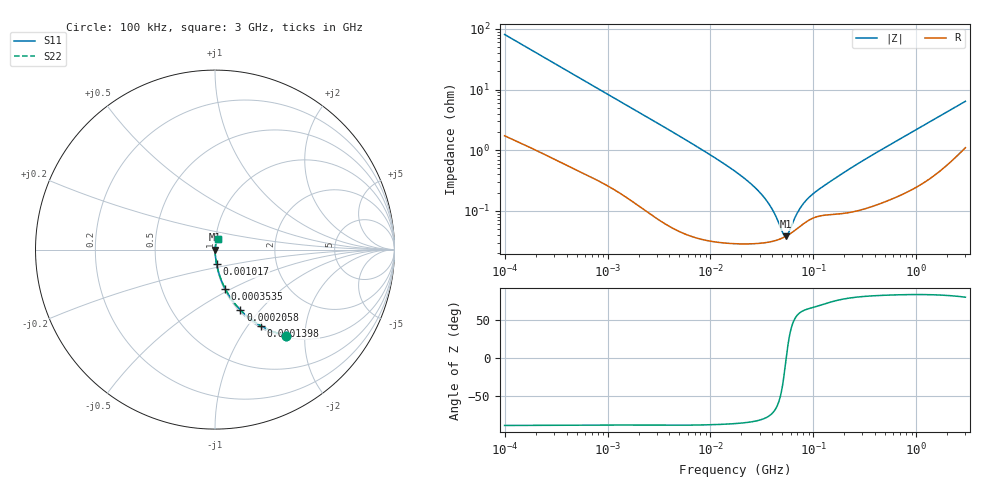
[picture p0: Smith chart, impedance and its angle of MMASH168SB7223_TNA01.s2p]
! MMASH168SB7223_TNA01  S-PARAMETER MODEL  ( Standard Model )
! Model Generated by TAIYO YUDEN Corporation (http://www.ty-top.com)
! Version 1.0
! TAIYO YUDEN Control No. 220601
! Copyright(c) 2013 TAIYO YUDEN CO.,LTD. All Rights Reserved.
! Product Description (link to TY-COMPAS)
! https://ds.yuden.co.jp/TYCOMPAS/or/detail?pn=MMASH168SB7223KTNA01&u=M
! Products Name : Multilayer Ceramic Capacitors
! Characteristics :
!  Capacitance : 0.022 [uF] , Rated Voltage : 100 [V] , TCC : X7R
!  Case Size : 1.6 x 0.8 / 0.063 x 0.031 [mm/inch] , Thickness : 0.8 / 0.031 [mm/inch]
!  (Conditions: Temperature = 25 [degC] , DC Bias Voltage = 0 [V])
! External Node Assignments :
!  1  o---| |---o  2
! GND o---------o GND
! Frequency Range : 100kHz  -  3GHz  [ 401 STEP ]
# MHZ S RI R 50
! Freq[MHz].  S11 Real  S11 Imag  S21 Real  S21 Imag  S12 Real  S12 Imag  S22 Real  S22 Imag
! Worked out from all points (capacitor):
!   401 points, 100 kHz to 3 GHz, reference 50 ohm
!   read as one part in series: C = 19.7 nF near 105.3 kHz
!   lowest |Z| = 38.2 mohm at 53.83 MHz (marker M1)
!   series resonance near 54.47 MHz, so ESL is about 430 pH
!   S11 on the Smith chart (normalised r, x): 100 kHz: 1.03, -1.61; 139.8 kHz: 1.03, -1.16; 205.8 kHz: 1.02, -0.79; 353.5 kHz: 1.01, -0.47; 1.017 MHz: 1.01, -0.17; 3 GHz: 1.02, +0.13
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0.1  0.3966 -0.4786  0.6034 0.4786  0.6034 0.4786  0.3966 -0.4786
0.1398  0.2566 -0.4254  0.7434 0.4254  0.7434 0.4254  0.2566 -0.4254
0.205778  0.1419 -0.3368  0.8581 0.3368  0.8581 0.3368  0.1419 -0.3368
0.353547  0.0567 -0.2182  0.9433 0.2182  0.9433 0.2182  0.0567 -0.2182
0.562235  0.0253 -0.1432  0.9747 0.1432  0.9747 0.1432  0.0253 -0.1432
1.017073  0.00927 -0.0816  0.9907 0.0816  0.9907 0.0816  0.00927 -0.0816
3.161081  0.00144 -0.027  0.9986 0.027  0.9986 0.027  0.00144 -0.027
9.331111  0.000404 -0.00897  0.9996 0.00897  0.9996 0.00897  0.000404 -0.00897
17.7727  0.000306 -0.00435  0.9997 0.00435  0.9997 0.00435  0.000306 -0.00435
25.49486  0.000294 -0.00266  0.9997 0.00266  0.9997 0.00266  0.000294 -0.00266
33.85116  0.000301 -0.00158  0.9997 0.00158  0.9997 0.00158  0.000301 -0.00158
40.54368  0.000317 -0.000957  0.9997 0.000957  0.9997 0.000957  0.000317 -0.000957
51.12795  0.000364 -0.000202  0.9996 0.000202  0.9996 0.000202  0.000364 -0.000202
53.83243  0.00038 -3.73e-05  0.9996 3.73e-05  0.9996 3.73e-05  0.00038 -3.73e-05
58.15973  0.00041 0.000207  0.9996 -0.000207  0.9996 -0.000207  0.00041 0.000207
67.88584  0.000494 0.000686  0.9995 -0.000686  0.9995 -0.000686  0.000494 0.000686
75.25761  0.000566 0.000993  0.9994 -0.000993  0.9994 -0.000993  0.000566 0.000993
85.60801  0.000664 0.00136  0.9993 -0.00136  0.9993 -0.00136  0.000664 0.00136
97.38194  0.000752 0.0017  0.9992 -0.0017  0.9992 -0.0017  0.000752 0.0017
210.9903  0.000944 0.0045  0.9991 -0.0045  0.9991 -0.0045  0.000944 0.0045
547.5153  0.00165 0.012  0.9984 -0.012  0.9984 -0.012  0.00165 0.012
3000  0.0147 0.0614  0.9853 -0.0614  0.9853 -0.0614  0.0147 0.0614
